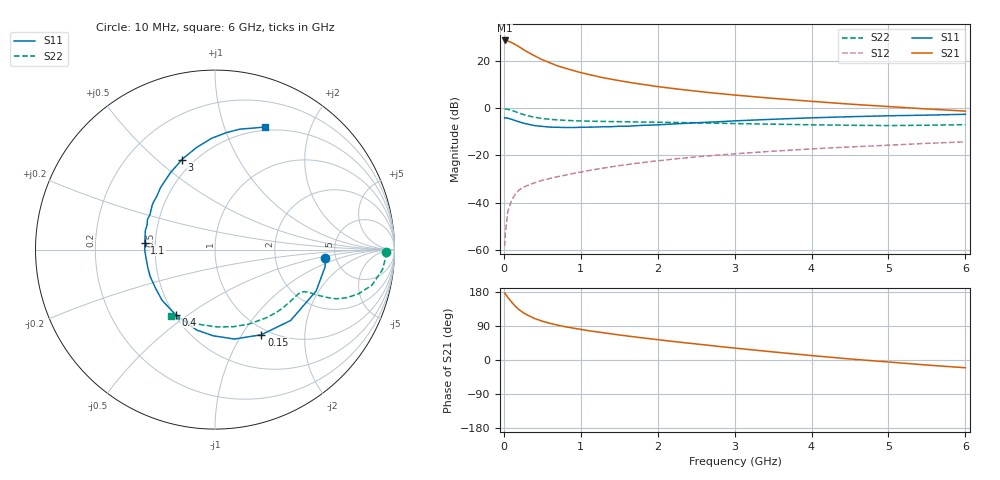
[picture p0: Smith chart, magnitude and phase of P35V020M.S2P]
! SIEMENS Small Signal Semiconductors
! BFP181
! Si NPN RF Bipolar Junction Transistor in SOT143
! VCE = 5 V  IC = 20 mA
! Common Emitter S-Parameters:  March  1996
# GHz  S  MA  R  50
!  f  S11  S21  S12  S22
! GHz  MAG  ANG  MAG  ANG  MAG  ANG  MAG  ANG
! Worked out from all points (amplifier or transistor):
!   36 points, 10 MHz to 6 GHz, reference 50 ohm
!   highest |S21| = 28.6 dB at 10 MHz (marker M1)
!   |S21| within 3 dB of that: start of sweep to 214.2 MHz
!   unconditionally stable (mu >= 1): start of sweep to 10.01286 MHz; 688.8 MHz to end of sweep
!   at 250 MHz: K = 0.52, MSG = 29.2 dB, |S12| = -33.6 dB
!   at 1.4 GHz: K = 1.23, MAG = 15.6 dB, |S12| = -24.8 dB
!   at 6 GHz: K = 1.02, MAG = 5.7 dB, |S12| = -14.3 dB
!   S11 on the Smith chart (normalised r, x): 10 MHz: 4.13, -0.60; 150 MHz: 0.91, -1.22; 400 MHz: 0.51, -0.45; 1.1 GHz: 0.44, +0.04; 3 GHz: 0.43, +0.61; 6 GHz: 0.46, +1.38
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0.01  0.6172 -4.2  26.79 176.6  0.0012 75.4  0.9547 -0.8
0.02  0.6207 -9.0  26.76 174.3  0.0023 86.2  0.9522 -2.5
0.05  0.609 -22.2  26.21 165.8  0.0063 84.8  0.9398 -6.8
0.1  0.5776 -43.1  24.15 153.0  0.0111 70.0  0.8964 -12.8
0.15  0.5402 -61.4  21.93 141.7  0.0152 65.1  0.8357 -17.2
0.2  0.51 -77.7  19.64 132.5  0.0187 61.7  0.7807 -20.1
0.25  0.4804 -91.1  17.36 125.1  0.0208 58.1  0.7317 -22.0
0.3  0.4599 -102.7  15.54 119.3  0.0228 56.1  0.6924 -22.9
0.4  0.424 -121.2  12.66 109.5  0.0263 54.6  0.6357 -23.8
0.5  0.4084 -136.3  10.48 102.4  0.0296 52.7  0.6 -24.2
0.6  0.3945 -147.7  9.006 96.8  0.0324 54.5  0.5759 -24.5
0.7  0.3911 -157.5  7.768 92.0  0.0354 54.6  0.559 -24.9
0.9  0.3867 -172.0  6.217 84.3  0.0414 55.0  0.5395 -26.0
1.1  0.3934 174.3  5.135 77.4  0.0476 55.7  0.5272 -27.7
1.3  0.4022 164.9  4.333 71.7  0.0539 55.6  0.5198 -29.9
1.5  0.4117 156.2  3.786 66.0  0.0606 55.5  0.5142 -32.1
2.2  0.4598 131.3  2.582 48.9  0.083 52.5  0.495 -42.3
3  0.5347 110.3  1.88 31.5  0.1076 47.0  0.469 -56.0
3.5  0.5783 100.2  1.599 21.3  0.1222 43.2  0.4554 -65.9
4.5  0.6545 84.5  1.208 2.7  0.1503 35.1  0.4311 -88.3
5.5  0.707 73.1  0.955 -13.3  0.1788 27.6  0.432 -111.8
6  0.7363 68.0  0.861 -20.5  0.1927 23.1  0.4447 -123.7
